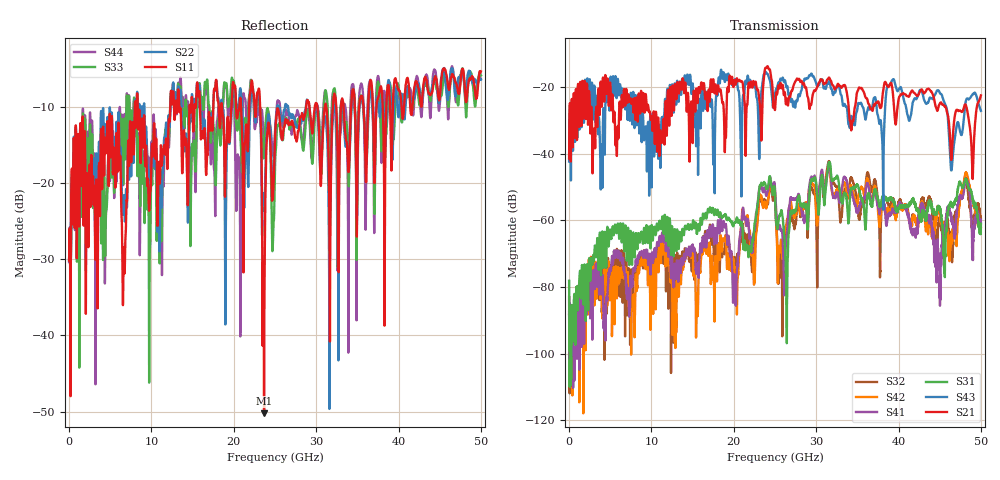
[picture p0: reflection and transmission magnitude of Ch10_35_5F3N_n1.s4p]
!Agilent Technologies,N5247A,US51170199,A.09.90.13
!Agilent N5247A: A.09.90.13
!Date: Tuesday, December 08, 2015 12:11:01
!Correction: S11(Full 4 Port(1,2,3,4))
!S12(Full 4 Port(1,2,3,4))
!S13(Full 4 Port(1,2,3,4))
!S14(Full 4 Port(1,2,3,4))
!S21(Full 4 Port(1,2,3,4))
!S22(Full 4 Port(1,2,3,4))
!S23(Full 4 Port(1,2,3,4))
!S24(Full 4 Port(1,2,3,4))
!S31(Full 4 Port(1,2,3,4))
!S32(Full 4 Port(1,2,3,4))
!S33(Full 4 Port(1,2,3,4))
!S34(Full 4 Port(1,2,3,4))
!S41(Full 4 Port(1,2,3,4))
!S42(Full 4 Port(1,2,3,4))
!S43(Full 4 Port(1,2,3,4))
!S44(Full 4 Port(1,2,3,4))
!S4P File: Measurements: <S11,S12,S13,S14>,
!<S21,S22,S23,S24>,
!<S31,S32,S33,S34>,
!<S41,S42,S43,S44>:
# Hz S  dB  R 50
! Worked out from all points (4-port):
!   3201 points, 10 MHz to 50 GHz, reference 50 ohm
!   strongest paths, dB at 10 MHz, 12.51 GHz, 25 GHz, 37.5 GHz, 50 GHz:
!     S21: -41.5, -21.7, -26.9, -24.3, -22.5
!     S43: -42.4, -19.4, -22.0, -28.6, -27.1
!     S31: -78.1, -62.0, -52.4, -53.6, -61.0
!     S41: -87.4, -72.0, -50.4, -55.3, -60.9
!     S42: -88.3, -80.2, -51.6, -56.8, -62.3
!     S32: -82.9, -69.1, -52.0, -54.4, -59.4
!   lowest |S11| = -50.2 dB at 23.68 GHz (marker M1), VSWR 1.01, Z = 50.1 + j0.297 ohm
!   |S11| at or under -10 dB: start of sweep to 7.973 GHz; 8.342 GHz to 12.29 GHz (3.946 GHz wide, 38.3 % of centre); 23.2 GHz to 28.79 GHz (5.586 GHz wide, 21.5 % of centre)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
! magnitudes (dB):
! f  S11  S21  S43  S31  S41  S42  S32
! 10 MHz  -30.2  -41.5  -42.4  -78.1  -87.4  -88.3  -82.9
! 18.6 GHz  -10.4  -24.7  -17.4  -59.2  -62.9  -68.2  -70.6
! 20.08 GHz  -7.4  -17.9  -18.2  -60.5  -77.3  -74.6  -71.0
! 23.68 GHz  -50.2  -16.9  -16.2  -48.5  -50.3  -54.7  -53.7
! 26.38 GHz  -11.8  -24.6  -20.1  -82.3  -65.4  -61.5  -63.3
! 31.57 GHz  -20.6  -17.2  -18.2  -42.5  -43.8  -44.0  -42.3
! 50 GHz  -5.4  -22.5  -27.1  -61.0  -60.9  -62.3  -59.4
